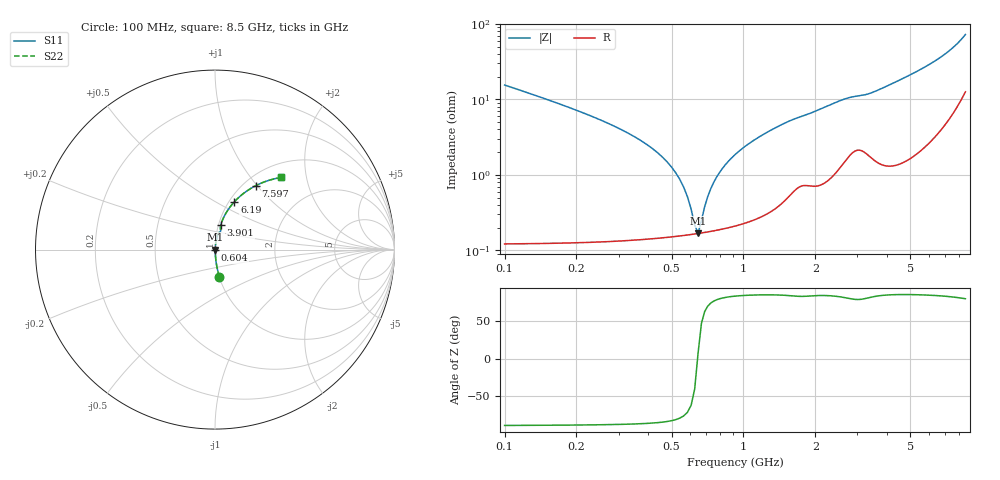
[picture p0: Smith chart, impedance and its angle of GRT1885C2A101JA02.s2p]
!Murata Part Number: GRT1885C2A101JA02
!These Parameters are Measured in Series Mode Connection
!Data Generated on Jun 19, 2026
!  o--ll--o
!Port1  Port2
!  o------o
!Operation Temp=25[degC], DC Bias Voltage=0[V]
!Freq. Start=100[MHz] Stop=9[GHz] 401[Steps]
# Hz S RI R 50
!Freq.(Hz) S11(Real) S11(Imag) S21(Real) S21(Imag) S12(Real) S12(Imag) S22(Real) S22(Imag)
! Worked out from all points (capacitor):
!   401 points, 100 MHz to 8.5 GHz, reference 50 ohm
!   read as one part in series: C = 100 pF near 142 MHz
!   lowest |Z| = 169 mohm at 646 MHz (marker M1)
!   series resonance near 643.1 MHz, so ESL is about 610 pH
!   S11 on the Smith chart (normalised r, x): 100 MHz: 1.00, -0.31; 604 MHz: 1.00, -0.01; 3.901 GHz: 1.03, +0.29; 6.19 GHz: 1.06, +0.62; 7.597 GHz: 1.13, +0.99; 8.5 GHz: 1.25, +1.43
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1e8  0.0247 -0.1513  0.9753 0.1513  0.9753 0.1513  0.0247 -0.1513
2.47e8  0.00428 -0.0546  0.9957 0.0546  0.9957 0.0546  0.00428 -0.0546
4.78e8  0.0017 -0.0149  0.9983 0.0149  0.9983 0.0149  0.0017 -0.0149
5.41e8  0.00162 -0.00859  0.9984 0.00859  0.9984 0.00859  0.00162 -0.00859
6.04e8  0.00163 -0.00311  0.9984 0.00311  0.9984 0.00311  0.00163 -0.00311
6.25e8  0.00164 -0.00141  0.9984 0.00141  0.9984 0.00141  0.00164 -0.00141
6.46e8  0.00167 0.000222  0.9983 -0.000222  0.9983 -0.000222  0.00167 0.000222
6.67e8  0.0017 0.00181  0.9983 -0.00181  0.9983 -0.00181  0.0017 0.00181
7.3e8  0.00182 0.0063  0.9982 -0.0063  0.9982 -0.0063  0.00182 0.0063
7.72e8  0.00192 0.00912  0.9981 -0.00912  0.9981 -0.00912  0.00192 0.00912
8.98e8  0.00233 0.0169  0.9977 -0.0169  0.9977 -0.0169  0.00233 0.0169
1.129e9  0.00347 0.0297  0.9965 -0.0297  0.9965 -0.0297  0.00347 0.0297
1.507e9  0.00707 0.0486  0.9929 -0.0486  0.9929 -0.0486  0.00707 0.0486
2.368e9  0.0169 0.0853  0.9831 -0.0853  0.9831 -0.0853  0.0169 0.0853
2.914e9  0.0308 0.1021  0.9692 -0.1021  0.9692 -0.1021  0.0308 0.1021
3.901e9  0.0329 0.1385  0.9671 -0.1385  0.9671 -0.1385  0.0329 0.1385
4.3e9  0.0395 0.1591  0.9605 -0.1591  0.9605 -0.1591  0.0395 0.1591
5.707e9  0.0836 0.2371  0.9164 -0.2371  0.9164 -0.2371  0.0836 0.2371
6.19e9  0.1081 0.2665  0.8919 -0.2665  0.8919 -0.2665  0.1081 0.2665
7.114e9  0.1762 0.3258  0.8238 -0.3258  0.8238 -0.3258  0.1762 0.3258
7.597e9  0.2276 0.3565  0.7724 -0.3565  0.7724 -0.3565  0.2276 0.3565
8.5e9  0.3676 0.4021  0.6324 -0.4021  0.6324 -0.4021  0.3676 0.4021
